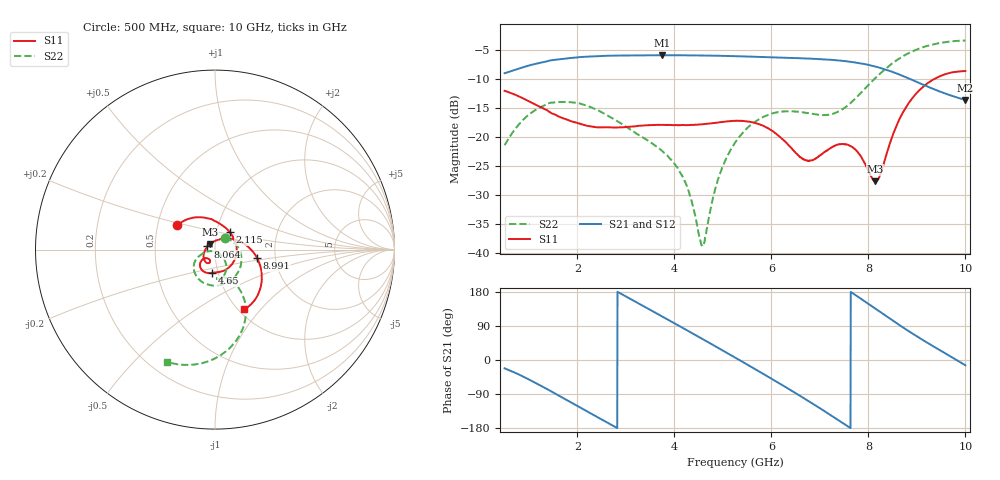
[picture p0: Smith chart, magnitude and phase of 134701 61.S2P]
!  2-Port S-parameters saved by WinCal
! VAR MeasName=S-Parameters (CALIBRATED_DATA) read from VNA (N5242A)
! VAR MeasDate=2013-7-3 16:41:12
! VAR NAME=134701 61
! VAR FILENAME=134701 61.S2P
! VAR DATE=2013-7-3 16:41:12
! VAR PHYS_PORTS=1,2
# Hz S MA R 50
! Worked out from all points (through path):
!   1601 points, 500 MHz to 10 GHz, reference 50 ohm
!   highest |S21| = -5.90 dB at 3.748 GHz (marker M1); lowest = -13.6 dB at 10 GHz (marker M2)
!   group delay of S21, straight-line fit = 210 ps
!   lowest |S11| = -27.6 dB at 8.136 GHz (marker M3), VSWR 1.09, Z = 47.2 + j2.87 ohm
!   |S11| at or under -10 dB: start of sweep to 9.358 GHz
!   |S22| runs from -38.8 to -3.4 dB; largest |S21 - S12| = 0.0018
!   S11 on the Smith chart (normalised r, x): 500 MHz: 0.63, +0.18; 2.115 GHz: 1.15, +0.23; 4.65 GHz: 0.94, -0.25; 8.064 GHz: 0.92, +0.03; 8.991 GHz: 1.60, -0.16; 10 GHz: 1.06, -0.82
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5e8  0.2502 147.5  0.355 -22.0  0.3549 -22.0  0.08507 49.5
9.809375e8  0.2052 118.7  0.411 -50.1  0.411 -50.1  0.1536 -17.1
1.45e9  0.1621 92.2  0.4576 -82.0  0.4576 -82.1  0.1976 -66.0
2.085312e9  0.129 52.7  0.4892 -127.3  0.4893 -127.3  0.1926 -113.7
2.115e9  0.1278 50.6  0.4903 -129.4  0.4899 -129.5  0.191 -115.6
2.875e9  0.1214 -11.1  0.5038 176.6  0.5037 176.6  0.1328 -148.5
3.670625e9  0.1273 -64.0  0.5072 120.4  0.5069 120.4  0.08056 -160.8
3.747812e9  0.1274 -67.8  0.5072 114.9  0.5071 114.9  0.07591 -161.9
4.222812e9  0.1268 -86.0  0.5065 81.1  0.506 81.1  0.0407 -166.6
4.555312e9  0.1287 -94.3  0.5042 57.1  0.5043 57.1  0.01184 -119.9
4.650312e9  0.1298 -96.5  0.5039 50.3  0.5037 50.2  0.01443 -72.2
4.911562e9  0.1338 -102.8  0.5015 31.3  0.5015 31.3  0.04467 -43.5
5.25e9  0.138 -112.3  0.4974 6.5  0.4978 6.4  0.08943 -49.9
5.6775e9  0.1318 -126.5  0.4912 -25.1  0.4923 -25.1  0.1368 -64.1
6.146562e9  0.1026 -139.9  0.4845 -60.3  0.4845 -60.4  0.164 -78.5
6.835312e9  0.06303 -120.3  0.4733 -113.9  0.4735 -113.9  0.1587 -85.4
7.55375e9  0.08612 -128.9  0.4486 -173.2  0.4495 -173.3  0.1841 -64.3
8.064375e9  0.04537 157.5  0.412 142.4  0.4127 142.3  0.2992 -58.8
8.135625e9  0.0415 132.9  0.4058 136.0  0.4057 136.0  0.3199 -59.5
8.420625e9  0.08259 48.5  0.3735 110.9  0.3728 110.9  0.4087 -65.3
8.990625e9  0.2383 -11.1  0.2997 63.2  0.2992 63.2  0.5664 -83.3
1e10  0.3706 -63.8  0.2089 -14.0  0.2088 -14.0  0.6791 -113.2
